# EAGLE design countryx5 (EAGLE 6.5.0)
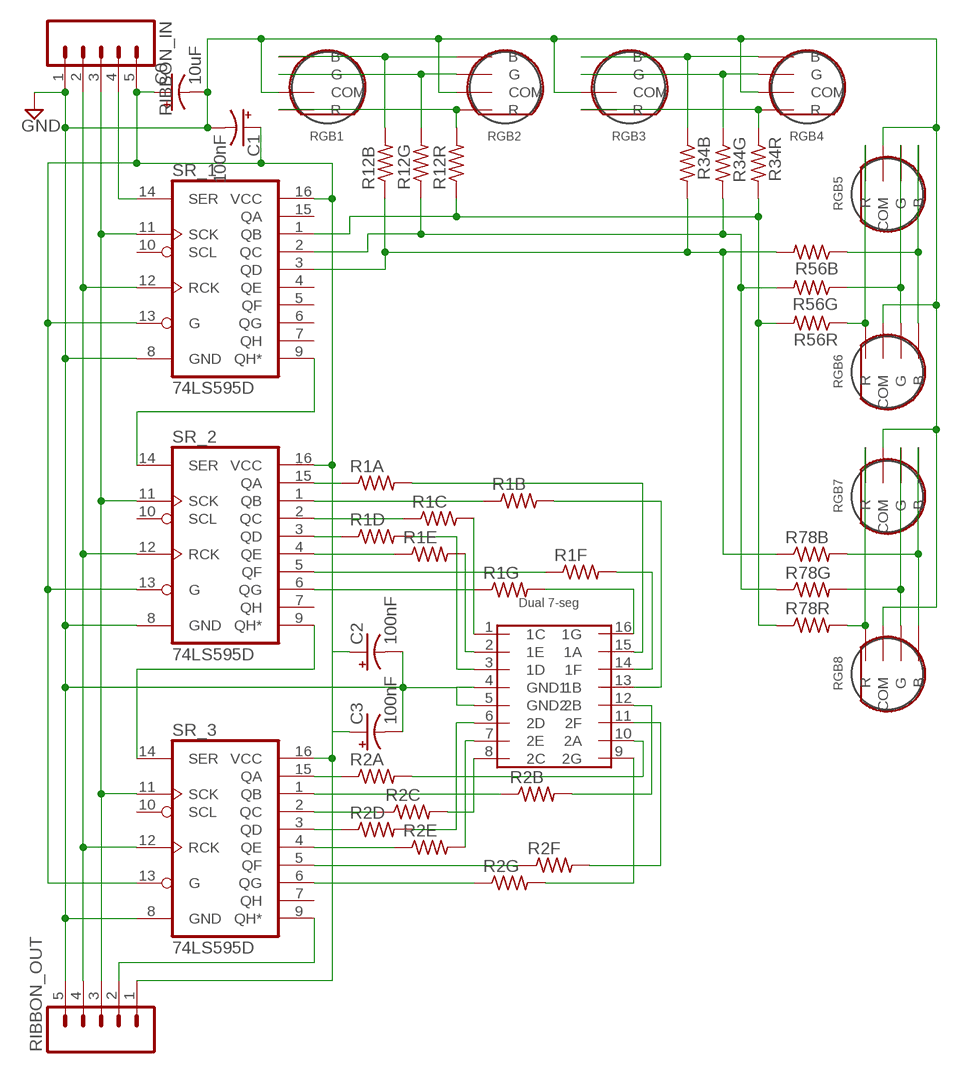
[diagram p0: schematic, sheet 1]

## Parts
C0  10uF  CAP_POL1206  [EIA3216]
C1  100nF  CAP_POL1206  [EIA3216]
C2  100nF  CAP_POL1206  [EIA3216]
C3  100nF  CAP_POL1206  [EIA3216]
R1A  R-US_M0805  [M0805]
R1B  R-US_M0805  [M0805]
R1C  R-US_M0805  [M0805]
R1D  R-US_M0805  [M0805]
R1E  R-US_M0805  [M0805]
R1F  R-US_M0805  [M0805]
R1G  R-US_M0805  [M0805]
R2A  R-US_M0805  [M0805]
R2B  R-US_M0805  [M0805]
R2C  R-US_M0805  [M0805]
R2D  R-US_M0805  [M0805]
R2E  R-US_M0805  [M0805]
R2F  R-US_M0805  [M0805]
R2G  R-US_M0805  [M0805]
R12B  R-US_M0805  [M0805]
R12G  R-US_M0805  [M0805]
R12R  R-US_M0805  [M0805]
R34B  R-US_M0805  [M0805]
R34G  R-US_M0805  [M0805]
R34R  R-US_M0805  [M0805]
R56B  R-US_M0805  [M0805]
R56G  R-US_M0805  [M0805]
R56R  R-US_M0805  [M0805]
R78B  R-US_M0805  [M0805]
R78G  R-US_M0805  [M0805]
R78R  R-US_M0805  [M0805]
RGB1  RGBLED  [3LED]
RGB2  RGBLED  [3LED]
RGB3  RGBLED  [3LED]
RGB4  RGBLED  [3LED]
RGB5  RGBLED  [3LED]
RGB6  RGBLED  [3LED]
RGB7  RGBLED  [3LED]
RGB8  RGBLED  [3LED]
RIBBON_IN  M05LOCK  [1X05_LOCK]
RIBBON_OUT  M05LOCK  [1X05_LOCK]
SR_1  74LS595D  [SO16]
SR_2  74LS595D  [SO16]
SR_3  74LS595D  [SO16]
U$1  HDSP-G03E  [HDSP-G]

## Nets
GND: C0.C(-) C1.C(-) C2.C(-) C3.C(-) RGB1.COM RGB2.COM RGB3.COM RGB4.COM RGB5.COM RGB6.COM RGB7.COM RGB8.COM RIBBON_IN.1 RIBBON_OUT.5 SR_1.8(GND) SR_2.8(GND) SR_3.8(GND) U$1.4(GND1) U$1.5(GND2)
N$1: R12R.1 R34R.2 R56R.2 R78R.1 SR_1.1(QB)
N$2: R12B.1 R34B.2 R56B.2 R78B.1 SR_1.3(QD)
N$3: R78R.2 RGB7.R RGB8.R
N$4: R1G.2 U$1.16(1G)
N$5: R1F.2 U$1.14(1F)
N$6: R1C.2 U$1.1(1C)
N$7: R1G.1 SR_2.6(QG)
N$8: R34B.1 RGB3.B RGB4.B
N$9: R1A.2 U$1.15(1A)
N$10: R1B.2 U$1.13(1B)
N$11: R2B.2 U$1.12(2B)
N$12: R2F.2 U$1.11(2F)
N$13: R2B.1 SR_3.1(QB)
N$14: R2D.2 U$1.6(2D)
N$15: R2A.1 SR_3.15(QA)
N$16: R1D.1 SR_2.3(QD)
N$17: R2E.2 U$1.7(2E)
N$18: R12R.2 RGB1.R RGB2.R
N$19: R2C.1 SR_3.2(QC)
N$20: R34R.1 RGB3.R RGB4.R
N$21: R2A.2 U$1.10(2A)
N$22: R2D.1 SR_3.3(QD)
N$23: R2E.1 SR_3.4(QE)
N$24: R2F.1 SR_3.5(QF)
N$25: R56B.1 RGB5.B RGB6.B
N$26: R12G.2 RGB1.G RGB2.G
N$27: R78B.2 RGB7.B RGB8.B
N$28: R12B.2 RGB1.B RGB2.B
N$31: R2G.1 SR_3.6(QG)
N$32: R12G.1 R34G.2 R56G.2 R78G.1 SR_1.2(QC)
N$33: R1E.1 SR_2.4(QE)
N$34: R34G.1 RGB3.G RGB4.G
N$37: R2G.2 U$1.9(2G)
N$38: R1E.2 U$1.2(1E)
N$42: R1F.1 SR_2.5(QF)
N$43: R56G.1 RGB5.G RGB6.G
N$45: R56R.1 RGB5.R RGB6.R
N$46: R78G.2 RGB7.G RGB8.G
N$48: R1D.2 U$1.3(1D)
N$52: R2C.2 U$1.8(2C)
N$53: R1C.1 SR_2.2(QC)
N$54: R1B.1 SR_2.1(QB)
N$55: R1A.1 SR_2.15(QA)
RCLK: RIBBON_IN.2 RIBBON_OUT.4 SR_1.12(RCK) SR_2.12(RCK) SR_3.12(RCK)
SCLK: RIBBON_IN.3 RIBBON_OUT.3 SR_1.11(SCK) SR_2.11(SCK) SR_3.11(SCK)
SER_12: SR_1.9(QH*) SR_2.14(SER)
SER_23: SR_2.9(QH*) SR_3.14(SER)
SER_IN: RIBBON_IN.4 SR_1.14(SER)
SER_OUT: RIBBON_OUT.2 SR_3.9(QH*)
VCC: C0.A(+) C1.A(+) C2.A(+) C3.A(+) RIBBON_IN.5 RIBBON_OUT.1 SR_1.13(G) SR_1.16(VCC) SR_2.13(G) SR_2.16(VCC) SR_3.13(G) SR_3.16(VCC)
Unconnected: SR_1.4(QE) SR_1.5(QF) SR_1.6(QG) SR_1.7(QH) SR_1.10(SCL) SR_1.15(QA) SR_2.7(QH) SR_2.10(SCL) SR_3.7(QH) SR_3.10(SCL)

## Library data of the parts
C0 C1-C3 = SparkFun-Capacitors:CAP_POL: Capacitor Polarized
R1A R1B R1C R1D R1E R1F R1G R2A R2B R2C R2D R2E R2F R2G R12B R12G R12R R34B R34G R34R R56B R56G R56R R78B R78G R78R = resistor:R-US_: RESISTOR, American symbol
RGB1-RGB8 = RISK:RGBLED
RIBBON_IN RIBBON_OUT = SparkFun-Connectors:M05: Header 5 Standard 5-pin 0.1" header. Use with straight break away headers (SKU : PRT-00116), right angle break away headers (PRT-00553), swiss pins (PRT-00743), machine pins (PRT-00117), and female headers (PRT-00115). Molex polarized connector foot print use with SKU : PRT-08230 with associated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
SR_1-SR_3 = SparkFun-DigitalIC:74*595: 8-bit SHIFT REGISTER, output latch; PROD_ID: IC-07875
U$1 = RISK:HDSP-G03E

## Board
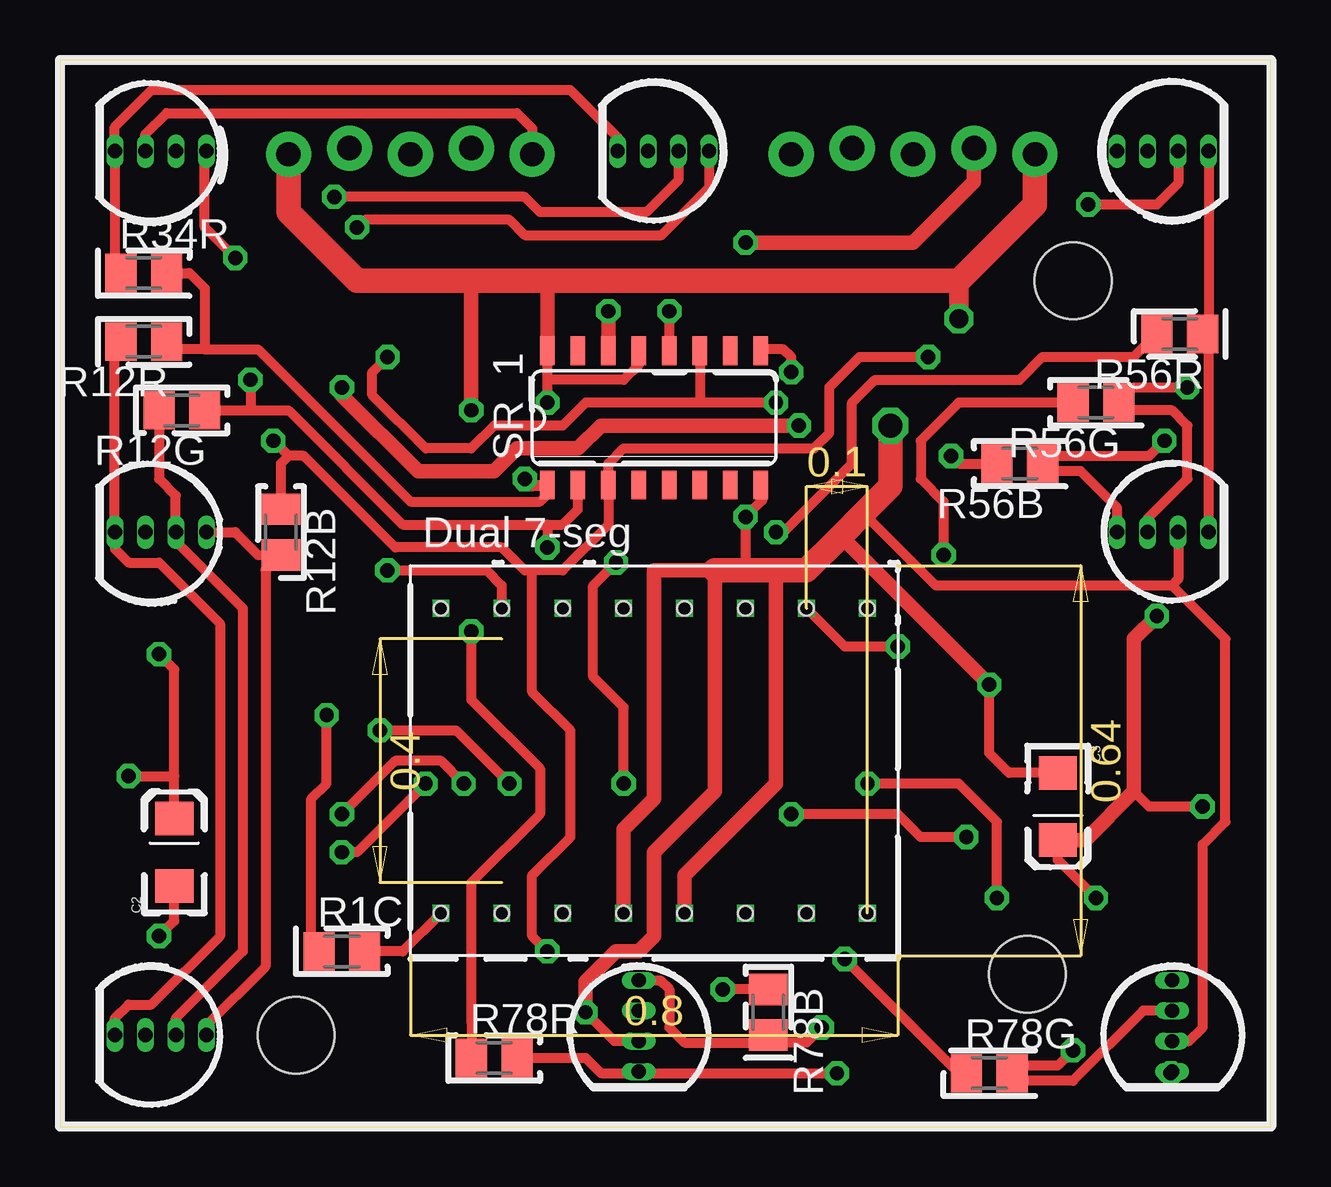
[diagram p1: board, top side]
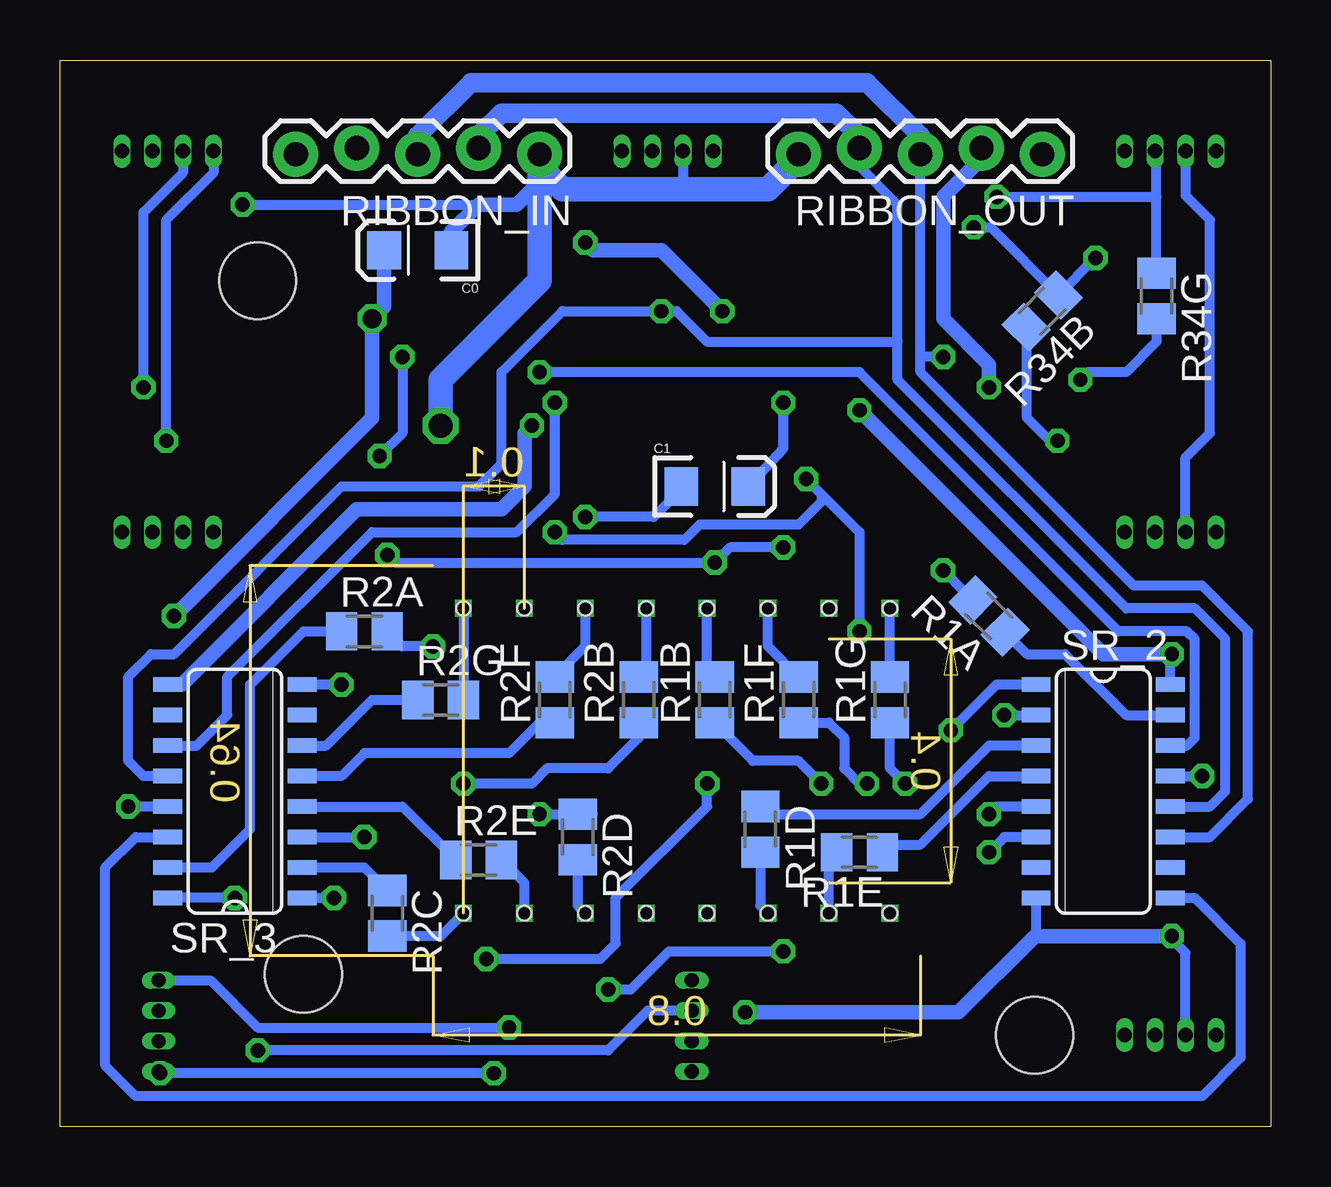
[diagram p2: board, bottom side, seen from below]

Size 50.47 x 44.44 mm. Coordinates in mm from the lower left corner, seen from the top.
Outline: 0,0 50.47,0 50.47,44.44 0,44.44 0,0
Copper layers (1*16): Top 0.035mm / dielectric 1.5mm / Bottom 0.035mm
Design rules "default *": minimum track width 10mil, minimum drill 24mil, track to track 8mil, track to pad 8mil, pad to pad 8mil, via to via 8mil, smd to smd 8mil, copper to edge 40mil, drill to drill 8mil, minimum pad ring 2mil, minimum via ring 8mil, stop-mask expansion 4mil, vias tented up to drill 0mil, thermal gap 10mil
Holes 3.2 mm at 40.32,6.35 9.84,3.81 42.23,35.24

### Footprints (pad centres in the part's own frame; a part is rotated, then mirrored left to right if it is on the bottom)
EIA3216 = smd 1.4 x 1.6: A 1.4,0; C -1.4,0
M0805 = smd 1.3 x 1.6: 1 -0.95,0; 2 0.95,0
3LED = drill 0.6 pad 0.61 long: B 0,2.286; COM 0,-0.254; G 0,1.016; R 0,-1.524
1X05_LOCK = drill 1.016 pad 1.88: 1 0,0.127; 2 2.54,-0.127; 3 5.08,0.127; 4 7.62,-0.127; 5 10.16,0.127
SO16 = smd 0.6 x 1.2: 1 -4.445,-2.8; 2 -3.175,-2.8; 3 -1.905,-2.8; 4 -0.635,-2.8; 5 0.635,-2.8; 6 1.905,-2.8; 7 3.175,-2.8; 8 4.445,-2.8; 9 4.445,2.8; 10 3.175,2.8; 11 1.905,2.8; 12 0.635,2.8; 13 -0.635,2.8; 14 -1.905,2.8; 15 -3.175,2.8; 16 -4.445,2.8
HDSP-G = drill 0.6 square: 1 -8.89,-6.35; 2 -6.35,-6.35; 3 -3.81,-6.35; 4 -1.27,-6.35; 5 1.27,-6.35; 6 3.81,-6.35; 7 6.35,-6.35; 8 8.89,-6.35; 9 8.89,6.35; 10 6.35,6.35; 11 3.81,6.35; 12 1.27,6.35; 13 -1.27,6.35; 14 -3.81,6.35; 15 -6.35,6.35; 16 -8.89,6.35 | hole 0.6: 1.27,-6.35; 1.27,-6.35; 1.27,-6.35; 1.27,-6.35; -1.27,-6.35; -1.27,-6.35; -3.81,-6.35; -3.81,-6.35; -6.35,-6.35; -6.35,-6.35; -6.35,-6.35; -8.89,-6.35; -8.89,-6.35; 3.81,-6.35; 3.81,-6.35; 3.81,-6.35; 6.35,-6.35; 6.35,-6.35; 8.89,-6.35; 8.89,-6.35; 8.89,-6.35; 8.89,6.35; 8.89,6.35; 6.35,6.35; 6.35,6.35; 3.81,6.35; 3.81,6.35; 1.27,6.35; 1.27,6.35; -1.27,6.35; -1.27,6.35; -3.81,6.35; -3.81,6.35; -6.35,6.35; -6.35,6.35; -6.35,6.35; -8.89,6.35; -8.89,6.35

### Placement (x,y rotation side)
C0  35.56,36.51 180 bottom
C1  23.18,26.67 0 bottom
C2  4.76,11.43 90 top
C3  41.59,13.34 270 top
R1A  11.75,21.27 135 bottom
R1B  23.18,17.78 90 bottom
R1C  11.75,7.3 0 top
R1D  21.27,12.38 270 bottom
R1E  17.14,11.43 180 bottom
R1F  19.68,17.78 90 bottom
R1G  15.88,17.78 90 bottom
R2A  37.78,20.64 0 bottom
R2B  26.35,17.78 90 bottom
R2C  36.83,8.89 270 bottom
R2D  28.89,12.06 270 bottom
R2E  33.02,11.11 0 bottom
R2F  29.84,17.78 90 bottom
R2G  34.61,17.78 0 bottom
R12B  9.21,24.77 270 top
R12G  5.08,29.84 180 top
R12R  3.49,32.7 180 top
R34B  9.53,33.97 225 bottom
R34G  4.76,34.61 270 bottom
R34R  3.49,35.56 0 top
R56B  40.01,27.62 180 top
R56G  43.18,30.16 180 top
R56R  46.67,33.02 180 top
R78B  29.53,4.76 270 top
R78G  38.73,2.22 0 top
R78R  18.1,2.86 0 top
RGB1  3.81,3.81 270 top
RGB2  3.81,24.77 270 top
RGB3  3.81,40.64 270 top
RGB4  24.77,40.64 270 top
RGB5  46.35,40.64 90 top
RGB6  46.35,24.77 90 top
RGB7  46.35,3.81 0 top
RGB8  24.13,3.81 0 top
RIBBON_IN  30.48,40.64 180 bottom
RIBBON_OUT  9.53,40.64 180 bottom
SR_1  24.77,29.53 0 top
SR_2  6.99,13.97 270 bottom
SR_3  43.18,13.97 90 bottom
U$1  24.77,15.24 0 top

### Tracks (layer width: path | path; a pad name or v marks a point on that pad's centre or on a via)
GND  (via drill 0.6, 1 pad 1.02)
  Top 0.406: v4.13,7.94 4.76,8.57 C2.C | C3.C 39.56,14.73 38.73,15.56 v38.73,18.41 | SR_1.8 29.27,26.67 29.27,26.09 v28.57,25.4 28.57,23.18 | RGB8.COM 23.11,3.56 v21.91,4.76 | RGB7.COM 47.05,3.56 47.62,4.13 47.62,11.75 48.58,12.7 48.58,20.32 46.35,22.54 | RGB6.COM 46.61,22.8 46.35,22.54 | 46.35,22.54 36.51,22.54 33.5,25.56 | RGB5.COM 46.61,39.31 45.72,38.42 v42.86,38.42 | RGB3.COM 3.56,41.34 4.45,42.23 19.05,42.23 19.68,41.59 RIBBON_OUT.5
  Top 0.61: U$1.5 26.04,10.48 29.84,14.29 29.84,23.18 | v38.73,18.41 32.54,24.61 | v21.91,4.76 21.91,6.03 23.18,7.3 24.13,7.3 24.77,7.94 24.77,11.43 27.3,13.97 27.3,23.18 24.77,23.18 24.77,13.65 23.5,12.38 U$1.4
  Top 1.016: 27.3,23.18 28.57,23.18 29.84,23.18 31.11,23.18 32.54,24.61 33.5,25.56 34.61,26.67 v34.61,29.21
  Bottom 0.406: RGB1.COM 3.56,7.24 4.13,7.81 v4.13,7.94 | SR_2.8 9.79,8.2 9.84,7.94 | RGB4.COM 24.51,38.8 24.45,39.05 | v38.73,18.41 SR_3.8 | v28.57,25.4 25.72,25.4 24.58,26.54 C1.C | v42.86,38.42 32.7,38.42 | RGB2.COM 3.56,27.88 2.54,28.89 2.54,37.78 3.56,38.8 RGB3.COM
  Bottom 0.61: v4.13,7.94 9.84,7.94 13.02,4.76 v21.91,4.76 | C0.C 34.16,37.28 33.02,38.42 32.7,38.42 31.43,38.42 30.16,39.69
  Bottom 1.016: RIBBON_OUT.5 19.68,40.32 20.95,39.05 24.45,39.05 29.53,39.05 30.16,39.69 30.48,40.01 RIBBON_IN.1 30.48,35.24 34.61,31.11 v34.61,29.21
N$1  (via drill 0.6 pad 1.02)
  Top 0.406: R34R.2 5.4,35.56 6.03,34.92 6.03,32.38 | R12R.1 4.76,32.38 6.03,32.38 | 6.03,32.38 8.26,32.38 14.61,26.04 20,26.04 20.32,26.35 20.32,26.67 | v17.14,20.64 17.14,17.78 20,14.92 20,13.02 17.14,10.16 17.14,5.71 R78R.1 | 20.32,26.67 19.68,26.67 v19.37,26.99 19.63,26.73 SR_1.1 20.32,26.67 | v29.84,24.77 30.16,24.77 33.02,27.62 33.02,30.16 33.97,31.11 40.01,31.11 40.96,32.07 44.77,32.07 R56R.2
  Bottom 0.406: 18.73,26.35 17.14,24.77 v17.14,20.64 | v19.37,26.99 18.73,26.35 | 18.73,26.35 18.73,26.04 19.68,25.08 23.81,25.08 24.45,24.45 29.53,24.45 v29.84,24.77
N$2  (via drill 0.6, 0.6 pad 1.02)
  Top 0.406: 19.68,23.18 20.95,23.18 22.86,25.08 SR_1.3 22.86,27.62 23.5,28.26 31.43,28.26 32.07,28.89 32.07,30.8 33.34,32.07 v36.2,32.07 | 19.68,23.18 19.68,18.1 21.27,16.51 21.27,12.06 19.68,10.48 19.68,7.94 v20.32,7.3 | 19.68,23.18 19.37,23.18 18.41,24.13 13.97,24.13 10.16,27.94 9.53,27.94 | R12B.1 9.21,27.62 9.53,27.94 | 9.53,27.94 v8.89,28.57 | R78B.1 27.94,5.72 v27.62,5.71 | v37.15,27.94 37.47,27.62 R56B.2
  Bottom 0.406: v8.89,28.57 9.21,28.57 10.16,29.53 10.16,33.26 R34B.2 | v27.62,5.71 26.67,5.71 25.08,7.3 v20.32,7.3 | v36.2,32.07 36.2,28.89 v37.15,27.94
N$3  (via drill 0.6)
  Top 0.406: 24.19,2.22 v32.38,2.22 | v46.29,2.23 RGB7.R | R78R.2 21.91,2.86 22.54,2.22 24.19,2.22 | 24.19,2.22 RGB8.R
  Bottom 0.406: v32.38,2.22 v46.29,2.23
N$4
  Bottom 0.406: R1G.2 U$1.16
N$5
  Bottom 0.406: R1F.2 20.95,20 U$1.14
N$6
  Top 0.406: U$1.1 14.29,7.3 R1C.2
N$7  (via drill 0.6)
  Top 0.406: v15.24,14.29 12.38,11.43 v11.75,11.43
  Bottom 0.406: SR_2.6 11.11,12.06 v11.75,11.43 | v15.24,14.29 15.88,14.92 R1G.1
N$8  (via drill 0.6)
  Top 0.406: RGB4.B 27.05,39.12 25.08,37.15 19.37,37.15 18.73,37.78 12.7,37.78 v12.38,37.47 | RGB3.B 6.03,40.58 6.03,37.47 v7.3,36.19
  Bottom 0.406: v7.3,36.19 R34B.1 11.67,37.47 v12.38,37.47
N$9  (via drill 0.6 pad 1.02)
  Top 0.406: v13.65,23.18 17.78,23.18 18.41,22.54 U$1.15
  Bottom 0.406: R1A.2 12.7,22.23 v13.65,23.18
N$10
  Bottom 0.406: R1B.2 23.5,19.05 U$1.13
N$11
  Bottom 0.406: U$1.12 26.04,19.05 R2B.2
N$12
  Bottom 0.406: U$1.11 28.57,20 R2F.2
N$13  (via drill 0.6)
  Top 0.406: v39.05,9.53 39.05,12.7 37.47,14.29 v33.66,14.29
  Bottom 0.406: R2B.1 26.35,16.19 27.62,14.92 30.16,14.92 30.8,14.29 v33.66,14.29 | SR_3.1 v39.05,9.53
N$14
  Bottom 0.406: R2D.2 28.89,9.21 U$1.6
N$15
  Bottom 0.406: SR_3.15 44.13,10.79 42.55,12.38 42.55,18.41 40.32,20.64 R2A.1
N$16
  Bottom 0.406: R1D.1 21.59,13.02 14.61,13.02 11.75,15.88 SR_2.3
N$17
  Bottom 0.406: U$1.7 31.11,10.16 R2E.2
N$18
  Top 0.406: RGB1.R 2.29,4.51 2.86,5.08 3.81,5.08 6.67,7.94 6.67,20.95 4.13,23.5 2.86,23.5 2.29,24.07 RGB2.R 2.29,32.45 R12R.2
N$19
  Bottom 0.406: SR_3.2 37.78,10.79 R2C.1
N$20
  Top 0.406: R34R.1 2.29,36.13 RGB3.R 2.29,41.66 3.81,43.18 21.27,43.18 23.24,41.21 RGB4.R
N$21  (via drill 0.6)
  Top 0.406: U$1.10 32.7,20 v34.92,20
  Bottom 0.406: v34.92,20 36.2,20 R2A.2
N$22  (via drill 0.6)
  Top 0.406: v37.78,12.06 35.88,12.06 34.92,13.02 v30.48,13.02
  Bottom 0.406: SR_3.3 v37.78,12.06 | v30.48,13.02 28.26,13.02 R2D.1
N$23
  Bottom 0.406: SR_3.4 36.19,13.34 R2E.1
N$24
  Bottom 0.406: SR_3.5 38.73,14.61 37.78,15.56 31.75,15.56 30.16,17.14 29.85,17.14 R2F.1
N$25  (via drill 0.6)
  Top 0.406: v46.04,28.57 45.4,27.94 41.27,27.94 R56B.1 41.59,27.3 42.55,27.3 44.07,25.78 RGB6.B
  Bottom 0.406: RGB5.B 44.07,39.75 46.04,37.78 v46.04,28.57
N$26
  Top 0.406: RGB1.G 4.83,4.51 7.62,7.3 7.62,21.59 4.83,24.38 RGB2.G 4.83,26.29 4.13,26.98 R12G.2
N$27  (via drill 0.6)
  Top 0.406: v31.75,4.13 31.11,3.49 29.84,3.49 R78B.2 29.21,3.49 26.04,3.49 25.4,4.13 25.4,5.71 25.02,6.1 RGB8.B
  Bottom 0.406: RGB7.B 44.2,6.1 42.23,4.13 v31.75,4.13
N$28
  Top 0.406: RGB1.B 6.1,4.19 8.57,6.67 8.57,23.18 R12B.2 8.26,23.81 7.3,24.77 RGB2.B
N$31
  Bottom 0.406: SR_3.6 39.37,15.88 37.47,17.78 R2G.1
N$32  (via drill 0.6, 0.6 pad 1.02)
  Top 0.406: R12G.1 7.94,29.84 | 7.94,29.84 9.53,29.84 14.29,25.08 20.32,25.08 | 20.32,25.08 20.95,25.08 21.59,25.72 SR_1.2 | v7.94,31.11 7.94,29.84 | R78G.1 37.47,2.22 v32.7,6.99 | v23.5,14.29 23.5,17.46 22.23,18.73 22.23,22.54 v23.18,23.5 | 20.32,25.08 v20.32,24.13 | R56G.2 37.47,30.16 35.88,28.57 35.88,26.99 36.83,26.04 v36.83,23.81
  Bottom 0.406: R34G.2 4.76,32.7 6.03,31.43 7.62,31.43 v7.94,31.11 | v32.7,6.99 27.94,6.99 27.3,7.62 27.3,9.53 23.5,13.34 v23.5,14.29 | v20.32,24.13 22.54,24.13 v23.18,23.5 36.51,23.5 v36.83,23.81
N$33
  Bottom 0.406: SR_2.4 11.75,14.61 14.61,11.74 16.2,11.74 R1E.1
N$34  (via drill 0.6)
  Top 0.406: RGB4.G 25.78,39.43 24.45,38.1 20,38.1 19.37,38.73 v11.43,38.73
  Bottom 0.406: R34G.1 4.76,38.73 | 4.76,38.73 4.76,40.58 RGB3.G | v11.43,38.73 4.76,38.73
N$37
  Bottom 0.406: U$1.9 R2G.2
N$38
  Bottom 0.406: U$1.2 18.41,11.11 R1E.2
N$42  (via drill 0.6)
  Top 0.406: v11.75,13.02 13.97,15.24 15.88,15.24 v16.83,14.29
  Bottom 0.406: SR_2.5 11.43,13.34 v11.75,13.02 | R1F.1 18.42,16.83 17.78,16.19 17.78,14.92 17.14,14.29 v16.83,14.29
N$43  (via drill 0.6)
  Top 0.406: RGB6.G 45.34,25.34 46.99,26.99 46.99,29.21 46.35,29.84 44.45,29.84 R56G.1 44.77,30.8 v46.99,30.8
  Bottom 0.406: RGB5.G 45.34,39.75 46.99,38.1 v46.99,30.8
N$45
  Top 0.406: RGB5.R 47.88,33.72 | 47.88,32.96 R56R.1 47.88,33.72 | RGB6.R 47.88,32.96 | 47.88,32.96 47.88,33.72
N$46  (via drill 0.6)
  Top 0.406: RGB7.G 45.15,4.83 42.23,1.91 40,1.91 R78G.2 40,2.54 41.59,2.54 v42.23,3.17
  Bottom 0.406: RGB8.G 25.97,4.83 27.62,3.17 v42.23,3.17
N$48
  Bottom 0.406: R1D.2 21.27,9.21 U$1.3
N$52
  Bottom 0.406: U$1.8 34.6,7.94 R2C.2
N$53  (via drill 0.6)
  Top 0.406: R1C.1 10.48,7.62 10.48,13.65 11.11,14.29 v11.11,17.14
  Bottom 0.406: v11.11,17.14 SR_2.2
N$54  (via drill 0.6)
  Top 0.406: v13.34,16.51 16.51,16.51 v18.73,14.29
  Bottom 0.406: SR_2.1 11.43,18.41 v13.34,16.51 | v18.73,14.29 19.68,15.24 21.59,15.24 21.91,15.56 R1B.1
N$55
  Bottom 0.406: SR_2.15 6.03,17.14 8.57,19.69 10.16,19.68 R1A.1
RCLK  (via drill 0.6)
  Top 0.406: SR_1.12 v25.4,33.97
  Bottom 0.406: SR_2.12 2.54,13.34 1.91,13.97 1.91,20.32 3.17,21.59 6.03,21.59 15.56,31.11 15.56,32.7 | 15.56,32.7 15.56,38.42 17.14,40.01 RIBBON_OUT.4 | SR_3.12 46.99,14.61 47.62,15.24 47.62,18.73 46.67,19.68 45.72,19.68 38.73,26.67 33.02,26.67 32.07,27.62 32.07,31.43 29.53,33.97 v25.4,33.97 24.77,33.97 23.5,32.7 15.56,32.7
  Bottom 0.813: RIBBON_OUT.4 17.14,41.27 18.1,42.23 32.07,42.23 33.02,41.27 RIBBON_IN.2
SCLK  (via drill 0.6)
  Top 0.406: v29.84,30.16 26.67,30.16 | SR_1.11 26.67,30.16 | 26.67,30.16 21.91,30.16 20.95,29.21 18.1,29.21 17.14,28.26 15.24,28.26 13.02,30.48 13.02,31.43 v13.65,32.07
  Bottom 0.406: SR_2.11 2.54,12.06 0.95,13.65 0.95,20.64 2.86,22.54 5.71,22.54 14.61,31.43 14.61,32.07 | 14.61,32.07 RIBBON_OUT.3 | SR_3.11 44.77,15.88 43.5,17.14 43.5,18.73 37.47,24.77 31.43,24.77 29.84,26.35 v29.84,30.16 | v13.65,32.07 14.61,32.07
  Bottom 0.813: RIBBON_IN.3 35.56,41.27 33.34,43.5 16.83,43.5 14.61,41.27 RIBBON_OUT.3
SER_12  (via drill 0.6)
  Top 0.406: v30.48,31.43 30.48,32.07 30.16,32.38 29.27,32.38 SR_1.9
  Bottom 0.406: SR_2.14 3.49,15.88 3.17,16.19 3.17,20.32 3.49,20.64 6.35,20.64 17.14,31.43 v30.48,31.43
SER_23
  Bottom 0.406: SR_2.9 3.17,9.53 1.27,7.62 1.27,2.86 2.86,1.27 47.31,1.27 48.58,2.54 48.58,10.79 47.31,12.06 SR_3.14
SER_IN  (via drill 0.6 pad 1.02)
  Top 0.61: SR_1.14 v22.86,33.97 | v28.57,36.83 35.56,36.83 38.1,39.37 RIBBON_IN.4
  Bottom 0.406: 28.26,36.51 v28.57,36.83
  Bottom 0.61: v22.86,33.97 25.4,36.51 28.26,36.51
SER_OUT  (via drill 0.6)
  Top 0.61: v11.75,30.8 11.75,30.48 14.92,27.3 18.1,27.3 19.05,28.26 21.59,28.26 22.54,29.21 v30.8,29.21
  Bottom 0.406: SR_3.9 45.4,18.41
  Bottom 0.61: RIBBON_OUT.2 12.06,40.32 13.65,38.73 13.65,33.66 11.75,31.75 v11.75,30.8 | v30.8,29.21 31.11,28.89 31.11,26.67 32.07,25.72 38.1,25.72 45.4,18.41
VCC  (via drill 0.6, 0.6 pad 1.02, 0.8 pad 1.02)
  Top 0.406: C2.A 4.76,14.61 | 4.76,14.61 4.76,19.05 v4.13,19.68 | v43.18,9.53 41.59,11.11 C3.A | v20.32,30.16 20.32,31.11 | 20.32,31.11 SR_1.16 | v2.86,14.61 4.76,14.61 | v47.62,13.34 45.4,13.34 44.77,13.97 | SR_1.13 24.13,31.75 23.5,31.11 20.32,31.11
  Top 0.61: SR_1.16 20.32,35.24 | v17.14,29.84 17.14,35.24 | C3.A 42.73,11.94 44.77,13.97 44.77,20.32 v45.72,21.27
  Top 0.813: 37.47,35.24 v37.47,33.66
  Top 1.016: RIBBON_OUT.1 9.53,38.1 12.38,35.24 17.14,35.24 20.32,35.24 37.47,35.24 40.64,38.42 RIBBON_IN.5
  Bottom 0.406: SR_2.16 4.18,19.63 v4.13,19.68 | v43.18,9.53 SR_3.16 | C1.A 20.32,28.26 v20.32,30.16 | SR_2.13 v2.86,14.61 | SR_3.13 v47.62,13.34
  Bottom 0.61: v4.13,19.68 6.99,19.68 v17.14,29.84 | v45.72,21.27 37.47,29.53 v37.47,33.66 36.96,34.16 C0.A

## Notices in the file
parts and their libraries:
SparkFun-DigitalIC: Licensing: Creative Commons ShareAlike 4.0 International - https://creativecommons.org/licenses/by-sa/4.0
